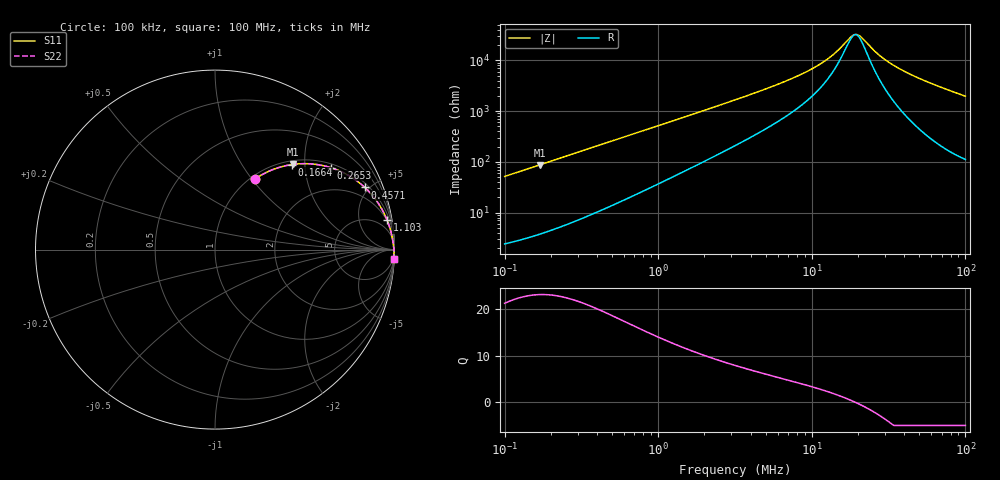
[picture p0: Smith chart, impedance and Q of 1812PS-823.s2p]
# MHz S MA R 50
!Freq  MagS11  AngS11  MagS21  AngS21  MagS12  AngS12  MagS22  AngS22
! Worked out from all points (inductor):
!   801 points, 100 kHz to 100 MHz, reference 50 ohm
!   read as one part in series: L = 81.9 uH near 103.5 kHz
!   highest Q = 23.2 at 169.3 kHz (marker M1), where L = 81.9 uH
!   self-resonance near 19.05 MHz
!   S11 on the Smith chart (normalised r, x): 100 kHz: 1.05, +1.03; 166.4 kHz: 1.07, +1.71; 265.3 kHz: 1.12, +2.73; 457.1 kHz: 1.24, +4.70; 1.103 MHz: 2, +11; 100 MHz: 3, -39
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0.1  0.4497 60.6  0.8723 -26.7  0.8723 -26.7  0.4497 60.6
0.166437  0.6376 48.0  0.7434 -39.6  0.7434 -39.6  0.6376 48.0
0.1693363  0.6439 47.5  0.7379 -40.0  0.7379 -40.0  0.6439 47.5
0.2653078  0.7904 35.3  0.5782 -52.1  0.5782 -52.1  0.7904 35.3
0.3180534  0.8364 30.7  0.5105 -56.7  0.5105 -56.7  0.8364 30.7
0.4570882  0.9037 22.5  0.3838 -64.5  0.3838 -64.5  0.9037 22.5
0.6569011  0.9439 16.2  0.2789 -70.4  0.2789 -70.4  0.9439 16.2
1.002882  0.969 10.8  0.1874 -75.1  0.1874 -75.1  0.969 10.8
1.102808  0.9726 9.8  0.171 -75.9  0.171 -75.9  0.9726 9.8
3.162278  0.9908 3.4  0.05962 -79.4  0.05962 -79.4  0.9908 3.4
6.419482  0.9944 1.5  0.0272 -77.4  0.0272 -77.4  0.9944 1.5
10.05773  0.9957 0.8  0.01455 -72.4  0.01455 -72.4  0.9957 0.8
13.25867  0.9963 0.4  0.008451 -63.8  0.008451 -63.8  0.9963 0.4
14.96236  0.9965 0.3  0.00613 -55.3  0.00613 -55.3  0.9965 0.3
17.78279  0.9968 0.1  0.003541 -25.4  0.003541 -25.4  0.9968 0.1
19.21985  0.9969 -0.0  0.003085 0.8  0.003085 0.8  0.9969 -0.0
20.77304  0.997 -0.1  0.003388 28.4  0.003388 28.4  0.997 -0.1
26.22708  0.9973 -0.4  0.006967 66.8  0.006967 66.8  0.9973 -0.4
31.71393  0.9974 -0.6  0.01088 76.0  0.01088 76.0  0.9974 -0.6
39.01665  0.9975 -0.9  0.01575 80.5  0.01575 80.5  0.9975 -0.9
50.11872  0.9975 -1.3  0.02263 83.0  0.02263 83.0  0.9975 -1.3
100  0.9958 -2.9  0.05066 83.8  0.05066 83.8  0.9958 -2.9
